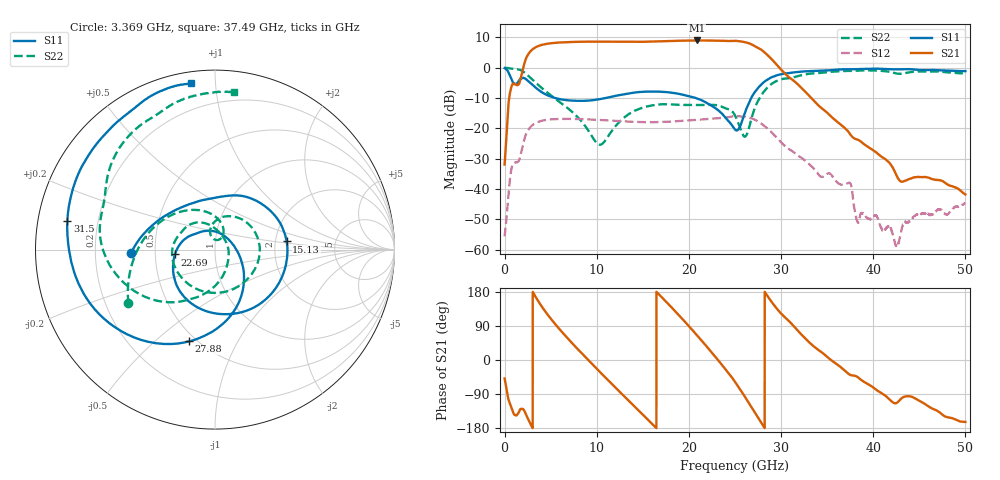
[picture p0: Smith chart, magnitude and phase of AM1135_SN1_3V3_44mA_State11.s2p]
!Agilent Technologies,E8364B,MY43040894,A.07.50.67
!Agilent E8364B: A.07.50.67
!Date: Monday, November 15, 2021 11:26:37
!Correction: S11(Full 2 Port(1,2))
!S21(Full 2 Port(1,2))
!S12(Full 2 Port(1,2))
!S22(Full 2 Port(1,2))
!S2P File: Measurements: S11, S21, S12, S22:
# Hz S  dB  R 50
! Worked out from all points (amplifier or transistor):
!   6401 points, 10 MHz to 50 GHz, reference 50 ohm
!   highest |S21| = 8.9 dB at 20.87 GHz (marker M1)
!   |S21| within 3 dB of that: 3.008 GHz to 27.83 GHz (24.83 GHz wide, 161 % of centre)
!   unconditionally stable (mu >= 1): start of sweep to end of sweep
!   at 8.336 GHz: K = 1.37, MAG = 9.1 dB, |S12| = -17.0 dB
!   at 25 GHz: K = 1.30, MAG = 9.1 dB, |S12| = -15.9 dB
!   at 50 GHz: K = 728.80, MAG = -30.3 dB, |S12| = -44.5 dB
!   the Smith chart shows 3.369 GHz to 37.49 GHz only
!   S11 on the Smith chart (normalised r, x): 3.369 GHz: 0.36, -0.02; 15.13 GHz: 2.31, +0.25; 22.69 GHz: 0.63, -0.04; 27.88 GHz: 0.46, -0.65; 31.5 GHz: 0.09, +0.10; 37.49 GHz: 0.06, +0.86
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1e7  -0.18 -10.5  -31.92 -48.8  -55.56 123.3  -0.05 -4.6
6.739297e8  -3.20 -58.7  -7.19 -120.6  -34.65 101.0  -0.29 -29.6
2.290794e9  -3.71 -130.5  2.68 -141.4  -22.26 57.1  -1.91 -104.4
3.368703e9  -6.59 -177.6  6.68 166.7  -18.26 3.3  -4.91 -148.1
5.665119e9  -10.14 134.7  8.20 89.9  -16.93 -71.5  -10.60 136.1
8.34427e9  -10.94 101.2  8.52 18.4  -16.96 -137.8  -17.66 69.8
1.003143e10  -10.54 83.3  8.57 -23.8  -17.18 -176.0  -24.92 71.8
1.199979e10  -9.33 59.3  8.54 -71.9  -17.53 141.3  -19.42 104.8
1.513198e10  -7.92 6.5  8.51 -147.2  -17.95 76.6  -13.04 51.2
1.667854e10  -7.90 -25.4  8.61 175.1  -17.92 44.9  -12.17 15.9
1.906088e10  -8.74 -80.2  8.85 114.5  -17.59 -5.6  -12.27 -48.6
2.08652e10  -10.13 -125.2  8.94 65.7  -17.19 -46.8  -12.34 -106.0
2.268515e10  -12.96 -173.1  8.90 14.1  -16.78 -91.3  -12.28 -164.1
2.5005e10  -20.37 76.2  8.84 -57.7  -15.95 -156.7  -15.76 113.2
2.626256e10  -13.40 -41.1  8.24 -103.8  -16.31 160.0  -22.14 -11.9
2.787942e10  -5.49 -105.8  5.84 -166.5  -18.48 100.2  -9.06 -124.6
2.925415e10  -2.83 -146.5  1.88 144.3  -22.10 55.0  -4.82 -167.4
3.149589e10  -1.53 169.0  -4.64 86.3  -28.14 3.8  -3.07 149.9
3.333927e10  -1.11 142.3  -10.19 40.4  -32.59 -36.6  -1.95 125.3
3.749469e10  -0.58 98.2  -21.92 -39.3  -38.04 -132.0  -1.08 82.9
4.167354e10  -0.52 58.0  -31.05 -101.9  -52.32 -122.1  -1.33 43.6
5e10  -1.15 -60.7  -41.75 -163.4  -44.52 -107.4  -1.58 -70.6
